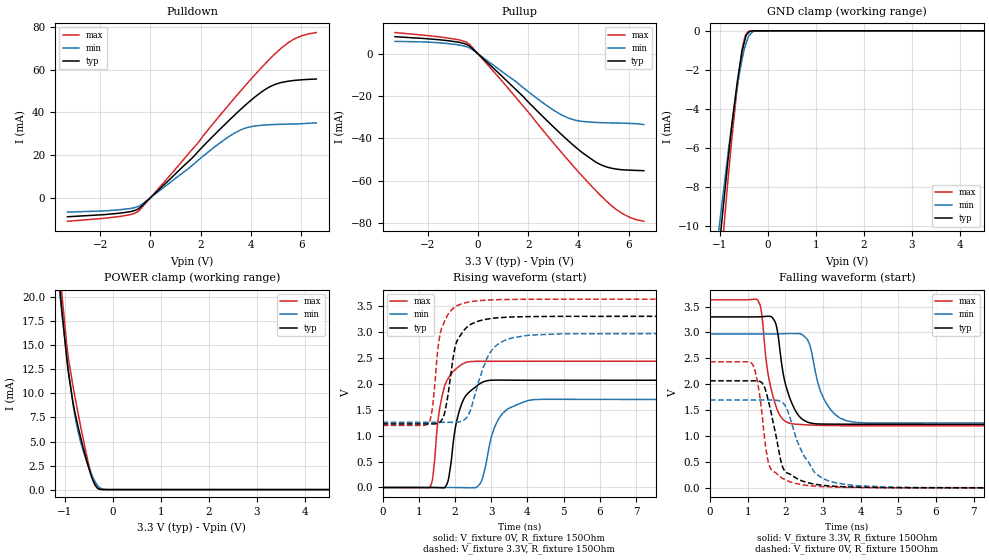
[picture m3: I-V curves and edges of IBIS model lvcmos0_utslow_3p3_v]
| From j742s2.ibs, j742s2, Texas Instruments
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|   utslow_3p3_v
[Model]   lvcmos0_utslow_3p3_v
Model_type   I/O
Polarity   Non-Inverting
Enable   Active-High
Vinl = 0
Vinh = 0.8
Vmeas = 1.65
Vref = 3.3
Cref = 2pF
Rref = 100000
|   typ   min   max
C_comp   1.414pF   1.380pF   1.447pF
[Voltage Range]   3.3   2.97   3.63
[Temperature Range]   27   150   -40
[Pullup Reference]   3.3   2.97   3.63
[Pulldown Reference]   0   0   0
[Power Clamp Reference]   3.3   2.97   3.63
[GND Clamp Reference]   0   0   0
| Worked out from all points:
|   slope of the pulldown table from 0 to 0.495 V, typ, clamps not added: 89.2 ohm
|   slope of the pullup table from 0 to 0.495 V, typ, clamps not added: 90.4 ohm
|   GND clamp passes 1 mA (typ) near -0.53 V on its own axis
|   POWER clamp passes 1 mA (typ) near -0.41 V on its own axis
|   falling waveform, V_fixture 3.3V, R_fixture 150Ohm: 20-80 % time 349ps typ, 425ps min, 302ps max; typ from 3.3 V to 1.23 V
|   rising waveform, V_fixture 0V, R_fixture 150Ohm: 20-80 % time 332ps typ, 421ps min, 279ps max; typ from 0 V to 2.07 V
|   rising waveform, V_fixture 3.3V, R_fixture 150Ohm: 20-80 % time 337ps typ, 523ps min, 276ps max; typ from 1.23 V to 3.3 V
|   falling waveform, V_fixture 0V, R_fixture 150Ohm: 20-80 % time 365ps typ, 617ps min, 269ps max; typ from 2.07 V to 0 V
[Pulldown]
|   Voltage   I(typ)   I(min)   I(max)
-3.3V     -8.928mA   -6.748mA   -11.05mA
-1.191V   -7.212mA   -5.619mA   -8.738mA
-498.3mV  -5.303mA   -4.129mA   -6.478mA
1.67V     18.72mA    15.24mA    22.76mA
2.779V    32.25mA    25.8mA     38.79mA
3.6V      41.52mA    31.84mA    50.21mA
4.036V    46.05mA    33.39mA    56.06mA
4.67V     51.5mA     34.18mA    64.09mA
5.125V    53.77mA    34.42mA    69.29mA
5.501V    54.67mA    34.52mA    72.83mA
6.026V    55.3mA     34.69mA    75.96mA
6.6V      55.65mA    35.07mA    77.43mA
[GND Clamp]
|   Voltage   I(typ)   I(min)   I(max)
-3.3V     -92.62mA   -62.37mA   -137.3mA
-1.558V   -24.44mA   -21.27mA   -28.6mA
-825mV    -6.576mA   -6.239mA   -7.571mA
-726mV    -4.419mA   -4.397mA   -5.03mA
-646.8mV  -2.874mA   -3.062mA   -3.168mA
-537.9mV  -1.081mA   -1.53mA    -1.069mA
-468.6mV  -411.8uA   -799.7uA   -249.5uA
-448.8mV  -221.6uA   -649.4uA   -177.7uA
-399.3mV  -88.3uA    -273.8uA   -22.85uA
-310.2mV  -2.821uA   -44.84uA   -952.2nA
-132mV    -55.92nA   -1.516uA   -88.26nA
6.6V      0A         0A         0A
[Pullup]
|   Voltage   I(typ)   I(min)   I(max)
-3.3V     8.073mA    5.863mA    10.01mA
-1.34V    6.388mA    4.989mA    7.694mA
-686.4mV  5.257mA    4.027mA    6.351mA
-349.8mV  3.728mA    2.82mA     4.582mA
996.6mV   -11.07mA   -8.755mA   -13.42mA
2.64V     -30.32mA   -23.62mA   -36.9mA
3.472V    -39.73mA   -29.7mA    -48.62mA
4.036V    -45.57mA   -31.73mA   -56.28mA
4.907V    -52.48mA   -32.52mA   -67.2mA
5.353V    -54.13mA   -32.66mA   -72.1mA
5.798V    -54.8mA    -32.77mA   -75.78mA
6.6V      -55.2mA    -33.44mA   -79.09mA
[POWER Clamp]
|   Voltage   I(typ)   I(min)   I(max)
-3.3V     165.9mA    145.4mA    188.3mA
-1.112V   21.57mA    20.89mA    23.69mA
-1.053V   18.36mA    18.1mA     20.07mA
-963.6mV  13.96mA    14.13mA    15.38mA
-914.1mV  11.87mA    12.11mA    13.39mA
-825mV    8.991mA    8.884mA    10.71mA
-735.9mV  6.868mA    6.368mA    8.325mA
-627mV    4.603mA    4.244mA    5.577mA
-468.6mV  1.77mA     1.94mA     2.021mA
-349.8mV  384.2uA    699uA      308.5uA
-290.4mV  89.89uA    295.9uA    37.18uA
6.6V      0A         0A         0A
[Ramp]
R_load = 150
|   typ   min   max
dV/dt_r   1.23976/3.29658e-10   1.01665/4.16925e-10   1.46005/2.78413e-10
dV/dt_f   1.24462/3.49036e-10   1.02857/4.20384e-10   1.46001/3.00932e-10
[Falling Waveform]
V_fixture = 3.3V
V_fixture_min = 2.97V
V_fixture_max = 3.63V
R_fixture = 150Ohm
C_fixture = 0F
|   Time   V(typ)   V(min)   V(max)
0s        3.3V       2.97V      3.63V
1.27ns    3.301V     2.97V      3.621V
1.365ns   3.304V     2.97V      3.388V
1.545ns   3.312V     2.97V      2.178V
1.725ns   3.207V     2.97V      1.634V
2.095ns   1.78V      2.979V     1.251V
2.575ns   1.273V     2.873V     1.216V
3.03ns    1.231V     1.706V     1.205V
3.635ns   1.229V     1.294V     1.2V
10ns      1.225V     1.255V     1.197V
[Rising Waveform]
V_fixture = 0V
V_fixture_min = 0V
V_fixture_max = 0V
R_fixture = 150Ohm
C_fixture = 0F
|   Time   V(typ)   V(min)   V(max)
0s        141.7uV    331.8uV    84.51uV
1.31ns    95.78uV    305.7uV    5.07mV
1.7ns     -6.73mV    169.4uV    1.923V
2.045ns   1.276V     -586.7uV   2.295V
2.28ns    1.748V     -3.299mV   2.404V
2.725ns   2.016V     112.1mV    2.432V
3.02ns    2.068V     1.011V     2.432V
3.315ns   2.069V     1.429V     2.432V
4.025ns   2.067V     1.677V     2.433V
10ns      2.066V     1.695V     2.434V
[Rising Waveform]
V_fixture = 3.3V
V_fixture_min = 2.97V
V_fixture_max = 3.63V
R_fixture = 150Ohm
C_fixture = 0F
|   Time   V(typ)   V(min)   V(max)
0s        1.225V     1.255V     1.197V
1.285ns   1.225V     1.256V     1.251V
1.61ns    1.277V     1.256V     3.018V
1.745ns   1.537V     1.256V     3.249V
2.005ns   2.711V     1.256V     3.481V
2.16ns    2.943V     1.272V     3.534V
2.385ns   3.12V      1.418V     3.574V
2.95ns    3.252V     2.581V     3.614V
3.43ns    3.281V     2.85V      3.623V
10ns      3.3V       2.97V      3.63V
[Falling Waveform]
|Gnd
V_fixture = 0V
V_fixture_min = 0V
V_fixture_max = 0V
R_fixture = 150Ohm
C_fixture = 0F
|   Time   V(typ)   V(min)   V(max)
0s        2.066V     1.695V     2.433V
1.125ns   2.066V     1.694V     2.388V
1.3ns     2.059V     1.694V     1.872V
1.57ns    1.617V     1.694V     437mV
1.905ns   453.1mV    1.657V     193.8mV
2.125ns   263.7mV    1.35V      116.9mV
2.39ns    149.8mV    772.9mV    67.71mV
2.75ns    75.06mV    326.5mV    35.41mV
3.31ns    30.4mV     102.7mV    15.3mV
10ns      140.3uV    332.5uV    84.44uV
